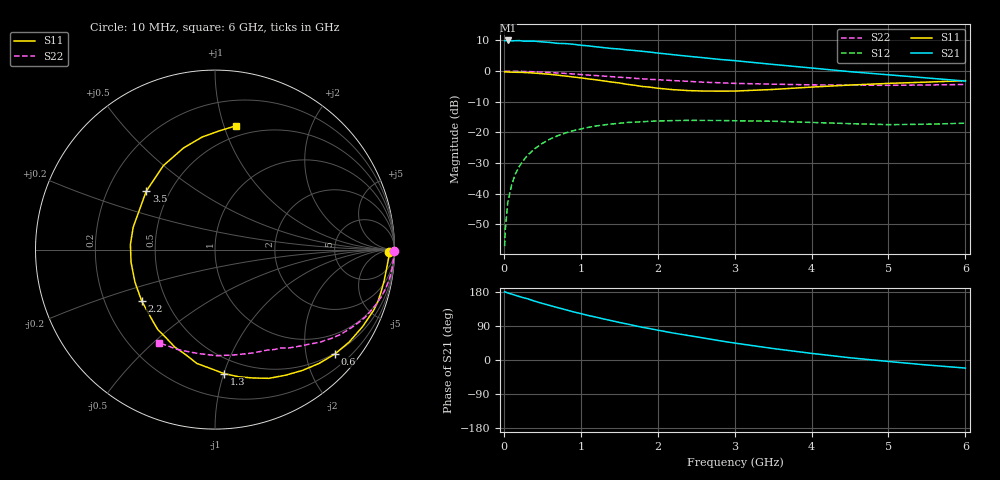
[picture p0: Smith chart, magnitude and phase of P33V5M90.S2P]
! SIEMENS Small Signal Semiconductors
! BFP181
! Si NPN RF Bipolar Junction Transistor in SOT143
! VCE = 3.5 V  IC = 0.9 mA
! Common Emitter S-Parameters:  March  1996
# GHz  S  MA  R  50
!  f  S11  S21  S12  S22
! GHz  MAG  ANG  MAG  ANG  MAG  ANG  MAG  ANG
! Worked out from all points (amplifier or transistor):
!   36 points, 10 MHz to 6 GHz, reference 50 ohm
!   highest |S21| = 10.0 dB at 50 MHz (marker M1)
!   |S21| within 3 dB of that: start of sweep to 1.572 GHz
!   unconditionally stable (mu >= 1): 3.257 GHz to end of sweep
!   at 250 MHz: K = 0.09, MSG = 19.5 dB, |S12| = -29.3 dB
!   at 1.4 GHz: K = 0.48, MSG = 12.3 dB, |S12| = -17.2 dB
!   at 6 GHz: K = 1.31, MAG = 3.5 dB, |S12| = -17.0 dB
!   S11 on the Smith chart (normalised r, x): 10 MHz: 53, -23; 600 MHz: 0.48, -2.60; 1.3 GHz: 0.38, -1.00; 2.2 GHz: 0.36, -0.28; 3.5 GHz: 0.37, +0.32; 6 GHz: 0.41, +1.10
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0.01  0.9687 -0.8  3.126 179.6  0.0014 79.3  0.9996 -0.3
0.02  0.972 -1.5  3.132 179.4  0.0027 89.2  0.9948 -0.6
0.05  0.9669 -3.4  3.162 176.9  0.0071 91.8  0.9971 -1.6
0.1  0.961 -7.0  3.114 174.0  0.0137 85.0  0.996 -3.2
0.15  0.958 -10.5  3.129 170.8  0.0212 82.4  0.9941 -4.9
0.2  0.9548 -14.1  3.149 167.6  0.0278 80.8  0.9916 -6.5
0.3  0.9469 -20.8  3.081 162.2  0.0415 76.3  0.9845 -9.7
0.4  0.9275 -27.6  3.075 155.3  0.0542 71.9  0.9755 -12.9
0.6  0.8863 -41.0  2.933 143.8  0.078 62.8  0.9484 -18.8
0.9  0.8026 -60.7  2.743 127.3  0.1065 50.5  0.8977 -26.8
1.1  0.746 -73.5  2.58 117.3  0.1213 43.7  0.8621 -31.5
1.3  0.6923 -85.9  2.415 108.2  0.1329 37.2  0.8293 -35.7
1.5  0.642 -99.1  2.298 99.2  0.1412 31.7  0.7955 -39.4
1.8  0.5616 -119.2  2.104 86.3  0.1499 24.7  0.7495 -44.5
2.2  0.4985 -145.1  1.854 71.2  0.156 16.2  0.7015 -50.7
2.8  0.4721 176.5  1.554 51.0  0.1567 7.1  0.647 -59.4
3  0.4726 164.7  1.482 44.7  0.1553 4.4  0.6313 -62.4
3.5  0.5026 139.7  1.286 30.3  0.1523 -0.1  0.613 -70.0
4  0.5493 121.6  1.124 17.5  0.1457 -3.3  0.5973 -79.0
4.5  0.593 107.2  0.98 5.9  0.1393 -4.8  0.5913 -89.2
5.5  0.6621 87.9  0.774 -13.2  0.1362 -1.3  0.5943 -110.3
6  0.699 80.5  0.688 -21.3  0.1417 0.1  0.6056 -121.2
